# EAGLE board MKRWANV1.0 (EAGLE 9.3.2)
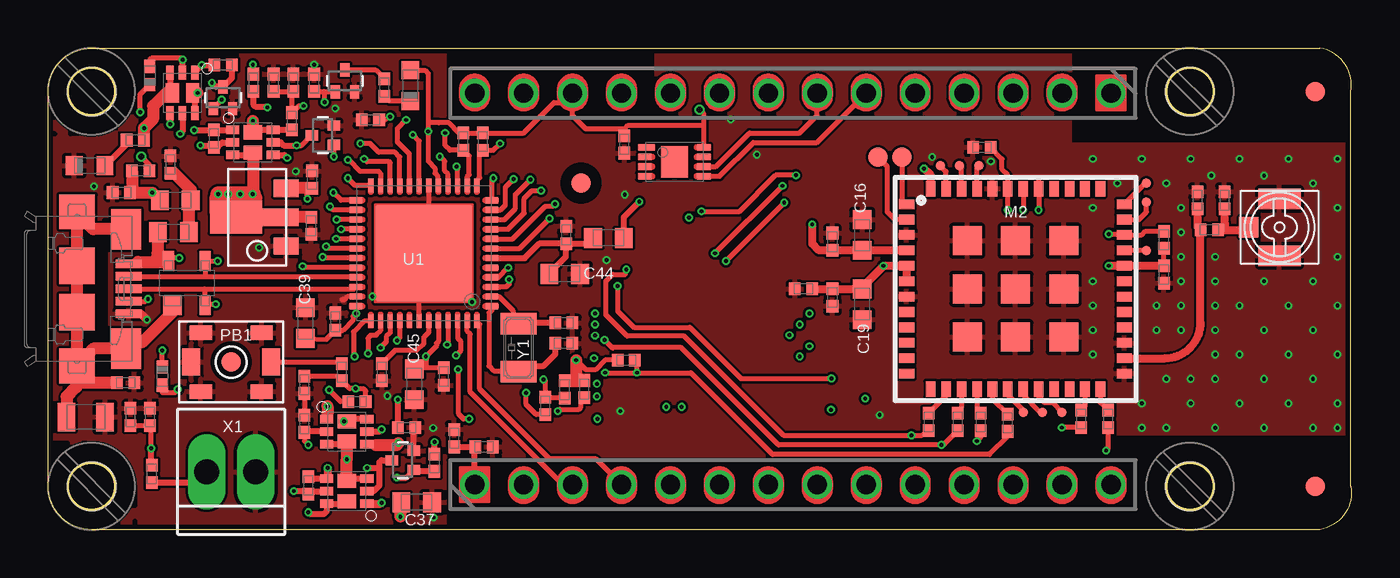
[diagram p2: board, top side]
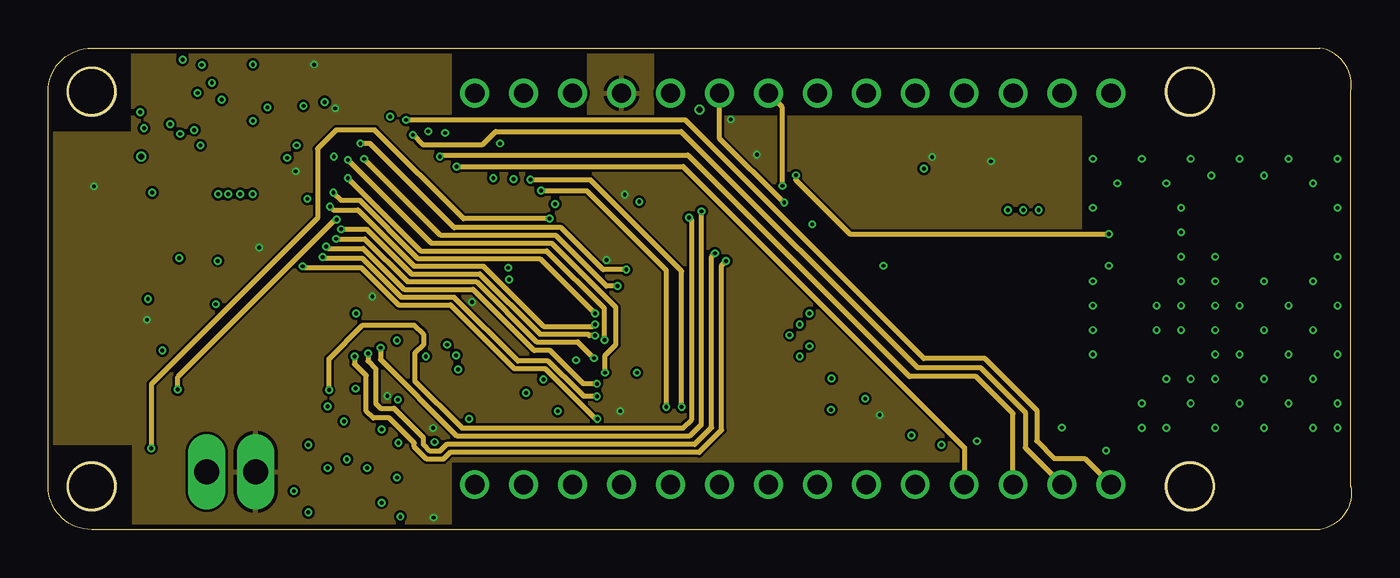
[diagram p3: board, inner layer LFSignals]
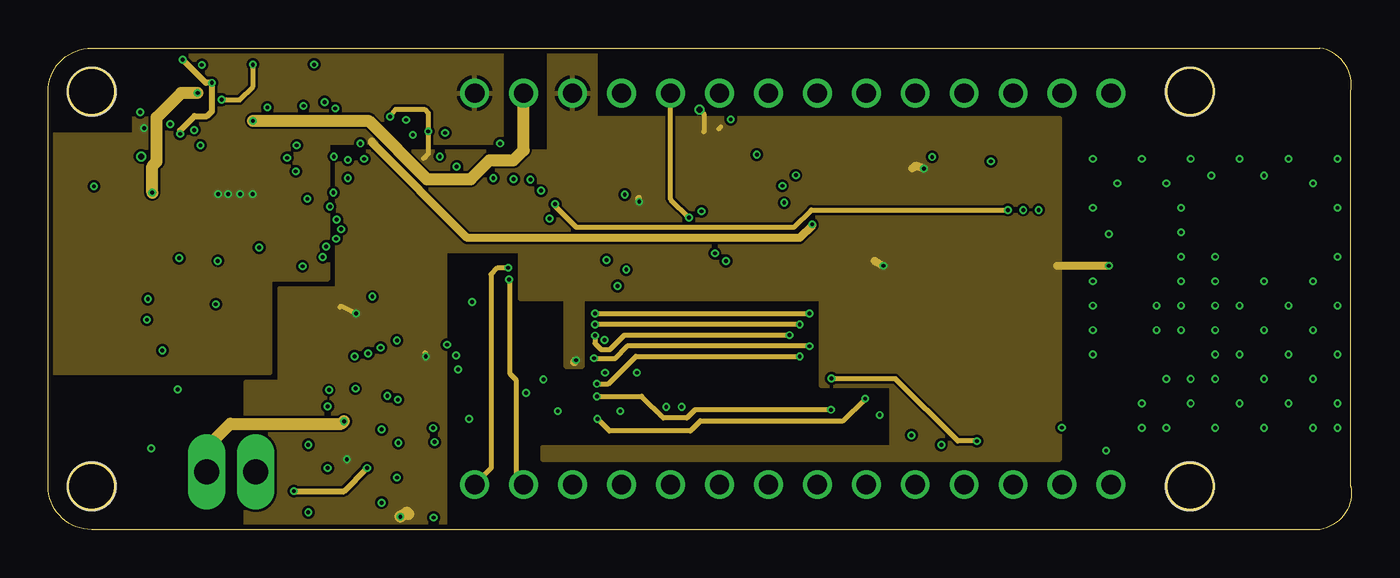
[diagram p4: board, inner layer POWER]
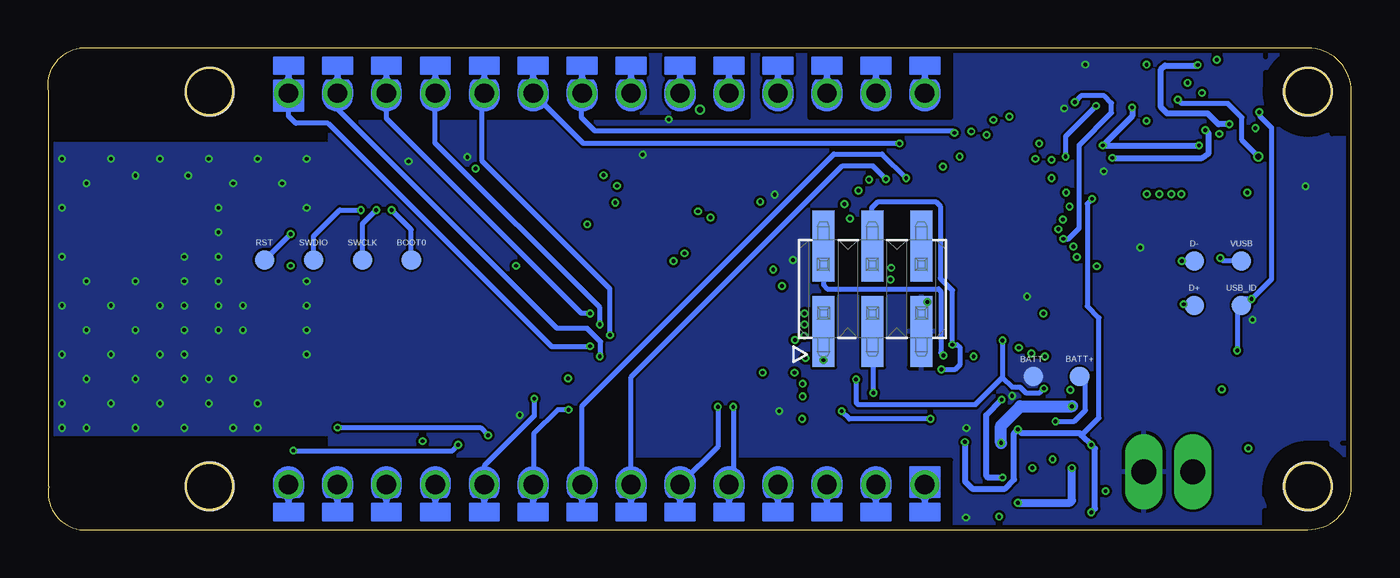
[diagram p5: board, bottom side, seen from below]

Size 67.63 x 25 mm. Coordinates in mm from the lower left corner, seen from the top.
Outline: 66,0 2.25,0 arc-90 0,2.25 0,22.75 arc-90 2.25,25 66,25 arc-90 67.6,22.75 67.6,2.25 arc-90 66,0
Copper layers (1*2*15*16): Top 0.035mm / dielectric 0.2mm / LFSignals 0.0175mm / dielectric 0.3mm / POWER 0.0175mm / dielectric 0.2mm / Bottom 0.035mm
Design rules "B&B_4layers *": minimum track width 8mil, minimum drill 0.195mm, track to track 5mil, track to pad 5mil, pad to pad 5mil, via to via 5mil, smd to smd 0mil, copper to edge 10mil, drill to drill 8mil, minimum pad ring 6mil, minimum via ring 4mil, stop-mask expansion 4mil, vias tented up to drill 25mil, thermal gap 7mil
Net classes: 0 default: width 0.25 mm, drill 0.195 mm
Holes 2.5 mm at 2.25,2.25 2.25,22.75 59.25,22.75 59.25,2.25
tRestrict: area 0,0 to 4.5,4.5; area 0,20.5 to 4.5,25; 18 lines
bRestrict: area 0,0 to 4.5,4.5; area 0,20.5 to 4.5,25; 18 lines

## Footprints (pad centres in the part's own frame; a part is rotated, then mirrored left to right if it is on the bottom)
TP-1.00MM = smd 1 x 1 bottom: X 0,0
0805-R2013X50N = smd 0.95 x 1.45: 1 -1,0; 2 1,0
0402-1005X55N = smd 0.62 x 0.62: 1 -0.45,0; 2 0.45,0
0603-1608X90N = smd 0.95 x 1: 1 -0.8,0; 2 0.8,0
SOT190P230X110-4N = smd 1 x 1: 1 -1.15,0.75 | smd 1 x 0.6: 2 -1.15,-0.95; 3 1.15,-0.95; 4 1.15,0.95
SODFL1008X40N-882D = smd 0.65 x 0.6: A 0.475,0; C -0.475,0
LEDC1608X80N-AK = smd 0.9 x 0.95: A 0.8,0; C -0.8,0
FD-1-1.5 = smd 1.016 x 1.016: P$1 0,0
ZX62-AB-5PA = smd 0.4 x 1.35: 1 -1.3,3.025; 2 -0.65,3.025; 3 0,3.025; 4 0.65,3.025; 5 1.3,3.025 | smd 2.1 x 1.6: 6 3.1,2.9; 11 -3.1,2.9 | smd 1.8 x 1.9: 7 4,0.35; 10 -4,0.35 | smd 1.9 x 1.9: 8 1.2,0.35; 9 -1.2,0.35
2X3_SMT = smd 1.143 x 3.683: 1 -2.54,-2.223; 2 -2.54,2.223; 3 0,-2.223; 4 0,2.223; 5 2.54,-2.223; 6 2.54,2.223
1X14_SMD_TH = drill 1: 1 0,0; 2 2.54,0; 3 5.08,0; 4 7.62,0; 5 10.16,0; 6 12.7,0; 7 15.24,0; 8 17.78,0; 9 20.32,0; 10 22.86,0; 11 25.4,0; 12 27.94,0; 13 30.48,0; 14 33.02,0
U.FL-R-SMT-1(60) = smd 1.05 x 2.2: GND1 -1.475,0; GND2 1.475,0 | smd 1.05 x 1: SIG 0,-1.6
0603-1608X90N@1 = smd 0.95 x 1: 1 -0.8,0; 2 0.8,0
CMWX1ZZABZ-078 = smd 0.8 x 0.5: 1 -5.65,4.4; 2 -5.65,3.6; 3 -5.65,2.8; 4 -5.65,2; 5 -5.65,1.2; 6 -5.65,0.4; 7 -5.65,-0.4; 8 -5.65,-1.2; 9 -5.65,-2; 10 -5.65,-2.8; 11 -5.65,-3.6; 12 -5.65,-4.4; 25 5.65,-4.4; 26 5.65,-3.6; 27 5.65,-2.8; 28 5.65,-2; 29 5.65,-1.2; 30 5.65,-0.4; 31 5.65,0.4; 32 5.65,1.2; 33 5.65,2; 34 5.65,2.8; 35 5.65,3.6; 36 5.65,4.4 | smd 0.5 x 0.8: 13 -4.4,-5.2; 14 -3.6,-5.2; 15 -2.8,-5.2; 16 -2,-5.2; 17 -1.2,-5.2; 18 -0.4,-5.2; 19 0.4,-5.2; 20 1.2,-5.2; 21 2,-5.2; 22 2.8,-5.2; 23 3.6,-5.2; 24 4.4,-5.2; 37 4.4,5.2; 38 3.6,5.2; 39 2.8,5.2; 40 2,5.2; 41 1.2,5.2; 42 0.4,5.2; 43 -0.4,5.2; 44 -1.2,5.2; 45 -2,5.2; 46 -2.8,5.2; 47 -3.6,5.2; 48 -4.4,5.2 | smd 1.5 x 1.5: 49 -2.5,2.5; 50 0,2.5; 51 2.5,2.5; 52 -2.5,0; 53 0,0; 54 2.5,0; 55 -2.5,-2.5; 56 0,-2.5; 57 2.5,-2.5
C&K_PTS820_NO_HOLES = smd 1.15 x 0.75: 1 -1.575,1.525; 2 -1.575,-1.525; 3 1.575,1.525; 4 1.575,-1.525 | smd 0.95 x 1.4: 5 -2.075,0; 6 2.075,0
PWR_SC70 = smd 0.69 x 0.4: D1 1.04,0.65; D2 -1.04,-0.65; G1 -1.04,0; G2 1.04,0; S1 -1.04,0.65; S2 1.04,-0.65 | smd 1 x 0.7: D1' 0,0.525; D2' 0,-0.525
SOTFL50P160X78-3 = smd 0.5 x 0.66: D 0,0.57; G -0.5,-0.57; S 0.5,-0.57
TP-0.50MM = smd 0.5 x 0.5 bottom: X 0,0
QFN50P700X700X90-49XN-EPSQ515 = smd 0.65 x 0.28: 1 -3.525,2.75; 2 -3.525,2.25; 3 -3.525,1.75; 4 -3.525,1.25; 5 -3.525,0.75; 6 -3.525,0.25; 7 -3.525,-0.25; 8 -3.525,-0.75; 9 -3.525,-1.25; 10 -3.525,-1.75; 11 -3.525,-2.25; 12 -3.525,-2.75; 25 3.525,-2.75; 26 3.525,-2.25; 27 3.525,-1.75; 28 3.525,-1.25; 29 3.525,-0.75; 30 3.525,-0.25; 31 3.525,0.25; 32 3.525,0.75; 33 3.525,1.25; 34 3.525,1.75; 35 3.525,2.25; 36 3.525,2.75 | smd 0.28 x 0.65: 13 -2.75,-3.525; 14 -2.25,-3.525; 15 -1.75,-3.525; 16 -1.25,-3.525; 17 -0.75,-3.525; 18 -0.25,-3.525; 19 0.25,-3.525; 20 0.75,-3.525; 21 1.25,-3.525; 22 1.75,-3.525; 23 2.25,-3.525; 24 2.75,-3.525; 37 2.75,3.525; 38 2.25,3.525; 39 1.75,3.525; 40 1.25,3.525; 41 0.75,3.525; 42 0.25,3.525; 43 -0.25,3.525; 44 -0.75,3.525; 45 -1.25,3.525; 46 -1.75,3.525; 47 -2.25,3.525; 48 -2.75,3.525 | smd 5 x 5: 49 0,0
SOT89-3L = smd 0.9 x 1.3: 1 -1.5,0; 3 1.5,0 | smd 0.9 x 1.9: 2 0,0.3 | smd 1.7 x 2.7: TH 0,2.6
SON50P300X200X60-9N-EP160X140 = smd 0.85 x 0.3: 1 -1.45,0.75 | smd 0.7 x 0.3: 2 -1.525,0.25; 3 -1.525,-0.25; 4 -1.525,-0.75; 5 1.525,-0.75; 6 1.525,-0.25; 7 1.525,0.25; 8 1.525,0.75 | smd 1.4 x 1.6: 9 0,0
SCREW2 = drill 1.3 long: GND 1.27,0; V+ -1.27,0
ABS07 = smd 1.1 x 1.9: 1 -1.25,0; 2 1.25,0

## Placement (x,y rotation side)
BATT+  DNP  [TP-1.00MM]  14.1,7.96 0 top
BATT-  DNP  [TP-1.00MM]  16.5,7.95 0 top
BOOT0  DNP  [TP-1.00MM]  48.78,14 0 top
C1  4n7  [0805-R2013X50N]  1.95,5.85 0 top
C2  10n  [0402-1005X55N]  6.35,18.95 90 top
C3  100n  [0402-1005X55N]  13.3,7.53 270 top
C4  20p  [0402-1005X55N]  26.76,9.67 180 top
C5  20p  [0402-1005X55N]  26.76,10.73 180 top
C6  100n  [0402-1005X55N]  3.8,17.5 180 top
C7  4u7  [0402-1005X55N]  21.07,4.75 90 top
C8  100n  [0402-1005X55N]  4.28,5.85 90 top
C9  100n  [0402-1005X55N]  22.62,4.3 0 top
C10  DNP  [0402-1005X55N]  59.64,17.1 90 top
C11  100n  [0402-1005X55N]  29.9,20 270 top
C12  DNP  [0402-1005X55N]  61.04,17.1 90 top
C14  100n  [0402-1005X55N]  11.7,23.2 90 top
C15  1u  [0402-1005X55N]  13.65,15.78 270 top
C16  10u  [0603-1608X90N]  42.25,15.3 90 top
C17  1u  [0402-1005X55N]  13.7,18.18 90 top
C18  100n  [0402-1005X55N]  40.7,14.95 90 top
C19  10u  [0603-1608X90N]  42.25,11.7 270 top
C20  1u  [0402-1005X55N]  40.7,12.05 270 top
C21  100n  [0402-1005X55N]  39.2,12.5 180 top
C22  100n  [0402-1005X55N]  57.9,13.25 270 top
C37  10u  [0603-1608X90N]  19.12,1.43 0 top
C38  100n  [0402-1005X55N]  16.73,21.27 180 top
C39  10u  [0603-1608X90N]  13.35,10.72 90 top
C40  100n  [0402-1005X55N]  14.9,10.8 90 top
C42  100n  [0402-1005X55N]  20.52,7.95 270 top
C43  100n  [0402-1005X55N]  26.88,15.3 90 top
C44  10u  [0603-1608X90N]  26.81,13.28 0 top
C45  10u  [0603-1608X90N]  19,7.55 270 top
C47  1u  [0402-1005X55N]  17.32,8.18 270 top
D1  PRTR5V0U2X,215  [SOT190P230X110-4N]  7.2,12.8 90 top
D1+  DNP  [TP-1.00MM]  44.3,19.35 0 bottom
D1-  DNP  [TP-1.00MM]  43.05,19.35 0 bottom
D2  PMEG2005EL  [SODFL1008X40N-882D]  5.92,7.97 270 top
D3  PMEG2005EL  [SODFL1008X40N-882D]  5.28,23.57 90 top
D+  DNP  [TP-1.00MM]  8.15,11.65 0 top
D-  DNP  [TP-1.00MM]  8.15,13.95 0 top
DL1  YELLOW  [LEDC1608X80N-AK]  18.8,23.05 90 top
DL2  GREEN  [LEDC1608X80N-AK]  2.15,18.9 0 top
F1  PTC  [0603-1608X90N]  6.5,15.45 180 top
FD1  DNP  [FD-1-1.5]  27.65,18 90 top
FD2  DNP  [FD-1-1.5]  65.75,22.75 180 top
FD3  DNP  [FD-1-1.5]  65.75,2.25 90 top
FD4  DNP  [FD-1-1.5]  9.5,8.7 0 top
FRAME1  DNP  [FRAME]  0,0 0 top
FRAME2  DNP  [FRAME]  0,0 0 top
J1  USB-MICRO  [ZX62-AB-5PA]  1.15,12.5 270 top
J2  DNP  [2X3_SMT]  24.85,12.5 0 bottom
J3  DNP  [1X14_SMD_TH]  22.13,2.34 0 top
J5  DNP  [1X14_SMD_TH]  55.15,22.66 180 top
J7  UFL  [U.FL-R-SMT-1(60)]  63.9,15.7 270 top
L1  FERRITE-470R  [0603-1608X90N@1]  6.6,17.1 180 top
L5  FERRITE-470R  [0603-1608X90N@1]  29.07,15.14 180 top
M2  CMWX1ZZABZ-078  [CMWX1ZZABZ-078]  50.2,12.5 0 top
PB1  RESET  [C&K_PTS820_NO_HOLES]  9.5,8.7 0 top
Q1  DMP2160UFDB  [PWR_SC70]  6.97,22.68 270 top
Q2  DMP2160UFDB  [PWR_SC70]  10.62,20.1 0 top
Q3  2N7002T  [SOTFL50P160X78-3]  14.25,20.48 90 top
Q4  2N7002T  [SOTFL50P160X78-3]  9.07,22.43 0 top
Q5  DMP2160UFDB  [PWR_SC70]  15.5,2 180 top
Q6  DMP2160UFDB  [PWR_SC70]  15.5,5.1 0 top
Q7  2N7002T  [SOTFL50P160X78-3]  18.4,3.6 90 top
Q8  2N7002T  [SOTFL50P160X78-3]  15.4,23.3 0 top
R1  1M  [0402-1005X55N]  4.03,7.62 180 top
R2  330R  [0402-1005X55N]  25.8,6.42 90 top
R3  330R  [0402-1005X55N]  15.25,8.18 270 top
R4  10k  [0402-1005X55N]  27.82,7.3 90 top
R5  10k  [0402-1005X55N]  26.8,7.28 90 top
R6  330R  [0402-1005X55N]  16.02,6.65 180 top
R7  330R  [0402-1005X55N]  17.45,22.95 270 top
R8  330k  [0402-1005X55N]  5.28,5.85 270 top
R9  680k  [0402-1005X55N]  5.38,2.9 270 top
R10  10k  [0402-1005X55N]  13.3,5.5 270 top
R11  10k  [0402-1005X55N]  13.5,2.3 90 top
R12  100k  [0402-1005X55N]  18.6,5.3 180 top
R13  47k  [0402-1005X55N]  20.05,3.48 90 top
R14  10k  [0402-1005X55N]  30,8.8 180 top
R16  10k  [0402-1005X55N]  57.9,15.05 270 top
R17  10k  [0402-1005X55N]  48.45,19.85 0 top
R18  DNP  [0402-1005X55N]  45.7,5.6 270 top
R19  DNP  [0402-1005X55N]  47.2,5.6 270 top
R20  0R  [0402-1005X55N]  48.4,5.6 270 top
R21  4k7  [0402-1005X55N]  21.55,20.15 90 top
R22  4k7  [0402-1005X55N]  22.55,20.15 90 top
R23  100k  [0402-1005X55N]  12.65,21.2 270 top
R24  100k  [0402-1005X55N]  12.72,23.2 270 top
R25  100k  [0402-1005X55N]  4.8,18.62 180 top
R26  330R  [0402-1005X55N]  10.65,23.2 90 top
R27  10k  [0402-1005X55N]  9.07,24.12 180 top
R28  10k  [0402-1005X55N]  8.6,20.3 90 top
R29  330R  [0402-1005X55N]  4.53,20.23 0 top
R30  0R  [0402-1005X55N]  60.26,15.56 0 top
R31  0R  [0402-1005X55N]  49.8,5.55 270 top
R32  0R  [0402-1005X55N]  53.6,5.75 270 top
R33  100k  [0402-1005X55N]  13.8,23.2 270 top
R34  0R  [0402-1005X55N]  55,5.75 270 top
RST  DNP  [TP-1.00MM]  56.4,14 0 top
SWCLK  DNP  [TP-1.00MM]  51.32,14 0 top
SWDIO  DNP  [TP-1.00MM]  53.86,14 0 top
TP1  DNP  [TP-0.50MM]  51.6,6.1 0 bottom
TP2  DNP  [TP-0.50MM]  50.6,6.1 0 bottom
TP3  DNP  [TP-0.50MM]  57,18 0 bottom
TP4  DNP  [TP-0.50MM]  57,17 0 bottom
TP5  DNP  [TP-0.50MM]  46.3,18.9 0 bottom
TP6  DNP  [TP-0.50MM]  47.3,18.9 0 bottom
TP7  DNP  [TP-0.50MM]  48.3,18.9 0 bottom
TP15  DNP  [TP-0.50MM]  57,14.5 0 bottom
TP18  DNP  [TP-0.50MM]  52.6,6.1 0 bottom
U1  D21G18  [QFN50P700X700X90-49XN-EPSQ515]  19.5,14.35 180 top
U2  LDO2SOT89-3L  [SOT89-3L]  12.35,16.23 90 top
U3  ECC508  [SON50P300X200X60-9N-EP160X140]  32.5,19.1 0 top
U$5  [MH_RND_F_2.2MM_NM]  2.25,2.25 90 top
U$6  [MH_RND_F_2.2MM_NM]  2.25,22.75 90 top
U$7  [MH_RND_F_2.2MM_NM]  59.25,22.75 90 top
U$8  [MH_RND_F_2.2MM_NM]  59.25,2.25 90 top
USB_ID  DNP  [TP-1.00MM]  5.7,11.65 0 top
VUSB  DNP  [TP-1.00MM]  5.7,13.95 0 top
X1  SCREW2X2.54  [SCREW2]  9.5,3 0 top
Y1  32.768KHz  [ABS07]  24.42,9.44 270 top

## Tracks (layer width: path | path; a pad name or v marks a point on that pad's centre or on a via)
+3V3  (via drill 0.2, 0.3)
  Top 0.25: 15.35,3.8 v15.5,3.65 | 20.8,21.12 20.27,21.12
  Top 0.254: 20.25,10.45 U1.44 20.25,9.78 20.15,9.68 20.15,9.55 v19.6,9 19.6,8.4 | 20.25,18.1 U1.17 20.23,18.32 20.07,18.5 20.07,18.75 19.73,19.12 v19.73,20.68 19.73,21.2 | U1.36 v15.97,11.22 15.82,11.07 15.82,10.88 15.3,10.35 C40.1 14.43,9.88 C39.1 | C42.1 19.6,8.4 | 19.6,8.4 C45.1 | DL1.A 19.55,23.85 19.73,23.68 19.73,21.2 | C38.1 17.48,21.27 v17.75,21.45 | 20.8,21.12 21.32,20.6 R21.2 R22.2 24.68,20.6 26.25,22.18 26.73,22.18 J5.12 27.2,22.64 27.2,21.5 27.9,20.8 29.9,20.8 | R14.2 28.9,8.8 28.4,8.3 27.9,8.3 v27.4,8.8 | C22.1 R16.2 | U3.8 34.02,21 | 34.02,21 34.02,21.57 v33.8,21.8 | C11.1 29.9,20.8 | 29.9,20.8 30.1,21 34.02,21 | 20.27,21.12 19.8,21.12 19.73,21.2
  Top 0.305: Q5.D2 15.62,2.65 Q5.D2' | Q6.D2 15.38,4.45 Q6.D2' | L5.1 29.87,16.22 v30.68,17.02
  Top 0.406: M2.6 M2.5 v43.35,13.7 42.3,12.65 C19.1 C20.1 C21.1 | M2.48 45.8,18.4 v45.45,18.75 | v55.05,13.7 M2.32 C22.1
  Top 0.61: v27.4,8.8 27.4,7.75 27.35,7.72 | Q5.D2' v15.5,3.65 Q6.D2' | R5.2 27.35,7.72 | 27.35,7.72 27.8,7.72 R4.2 | C37.1 v18.27,0.68
  POWER 0.254: 19.48,19.27 19.73,19.52 v19.73,20.68 19.73,21.62 19.52,21.82 18.02,21.82 v17.75,21.45 | v15.97,11.22 15.2,11.6 15.15,11.55 | v19.6,9 19.6,9.12 19.55,9.18 | 34.8,20.8 34.9,20.9 | v33.8,21.8 34.02,21.57 34.02,20.65
  POWER 0.305: v30.68,17.02 30.62,17.2 30.65,17.23
  POWER 0.406: 27.3,8.7 v27.4,8.8 | v43.35,13.7 42.95,13.9 42.9,13.95 | v45.45,18.75 45,18.9 44.85,18.75 | v55.05,13.7 52.35,13.7
  POWER 0.61: v18.27,0.68 18.62,0.88 18.7,0.8
  Bottom 0.254: v27.4,8.8 27.4,10.27 J2.1
  pour POWER: 52.5,21.35 28.4,21.35 28.4,24.9 26,24.9 26,19.6 15,19.6 15,12.5 12,12.5 12,7.65 10.25,7.65 10.25,0.05 20.6,0.05 20.6,14.5 24.5,14.5 24.5,12 26.85,12 26.85,8.47 27.72,8.47 27.72,12 40.1,12 40.1,7.5 43.75,7.5 43.75,4.25 25.65,4.25 25.65,3.65 52.5,3.65
+5V  (via drill 0.2)
  Top 0.25: 8.7,17.55 v8.82,17.43
  Top 0.254: U2.TH U2.2
  Top 0.305: Q2.D2 10.5,19.45 Q2.D2' | Q1.D2 6.33,22.8 Q1.D2'
  Top 0.406: M2.4 C16.1 C18.1 40,14.5 39.65,14.85 v39.65,15.85
  Top 0.61: R29.2 v4.97,20.85 5.45,21.32 5.45,22 6.12,22.68 Q1.D2' | U2.TH 10.51,16.23 10.79,16.51 10.79,17.23 v10.61,17.43 10.62,17.45 Q2.D2' | 10.62,17.43 10.62,17.4 | 8.75,16.4 8.7,16.4 8.7,17.3 v8.82,17.43 | C15.1 U2.2
  Top 0.813: v8.82,17.43 v10.61,17.43 10.62,17.43
  POWER 0.406: 16.8,20.15 16.8,20.1 21.75,15.15 39,15.15 39.65,15.8 v39.65,15.85
  other vias: 9.34,17.43 9.97,17.43
  pour POWER: 23.5,25 23.5,20.1 14.5,20.1 14.5,13 11.5,13 11.5,8.15 0,8.15 0,20.5 4.5,20.5 4.5,25
GND  (via drill 0.2)
  Top 0.254: U1.18 19.75,14.6 U1.49 19.25,14.1 U1.42 | U1.35 15.53,12.1 15.38,11.95 15.28,11.95 15.25,11.93 | C3.2 R10.1
  Top 0.305: Q7.S 18.97,5.22 R12.1
  Top 0.406: J1.5 4.83,11.2 v5.12,10.9
  other vias: 43.15,5.95 56.75,6.55 58.02,7.82 66.91,9.09 60.56,5.28 58.02,5.28 63.1,5.28 65.64,5.28 66.91,5.28 28.98,14 29.93,17.4 16.82,12.1 22,11.82 10.95,14.65 19.98,5.28 20,0.62 12.85,18.6 14.9,21.88 13.8,24.15 2.38,17.82 36.77,19.48 17.6,6.94 45.88,19.35 48.92,19.12 60.56,10.36 65.64,10.36 54.21,11.63 54.21,16.71 54.21,19.25 55.48,17.98 56.75,19.25 58.02,17.98 60.36,18.38 63.1,18.38 65.64,17.98 59.29,19.25 61.83,19.25 64.37,19.25 66.91,19.25 66.91,16.71 66.91,14.17 60.56,12.9 60.56,14.17 63.1,12.9 65.64,12.9 61.83,11.63 64.37,11.63 66.91,11.63 63.1,10.36 61.83,9.09 64.37,9.09 65.64,7.82 63.1,7.82 60.56,7.82 59.29,6.55 61.83,6.55 64.37,6.55 66.91,6.55 29.69,6.15 58.79,12.9 58.79,14.17 58.79,10.36 58.79,11.63 59.29,7.82 57.52,10.36 57.52,11.63 60.56,11.63 58.79,15.44 58.79,16.71 54.21,10.36 54.21,9.09 54.21,12.9 60.56,9.09 56.75,5.28 35.42,21.3
  pour Bottom: 52.85,20 67.6,20 67.6,5 52.85,5
  pour Top: -1,25 53,25 53,0 -1,0
  pour Bottom: -1,25 53,25 53,0 -1,0
  pour Top (isolate 0.1): 52.88,20 67.6,20 67.6,5 52.88,5
  pour LFSignals: 0,4.5 0,20.55 4.45,20.55 4.45,25 20.8,25 20.8,21 28.1,21 28.1,25 31.3,25 31.3,21.4 53.52,21.4 53.52,5 53.52,3.6 20.8,3.6 20.8,0 4.5,0 4.5,4.5
N1  (via drill 0.2)
  Top 0.305: Q5.S2 13.6,2.65 R11.2
  Top 0.406: Q5.S1 17.25,1.35 v17.3,1.4 | v14.5,3.2 14.5,2.69 Q5.S2
  Bottom 0.406: v17.3,1.4 14.6,1.4 14.5,1.5 v14.5,3.2
N2  (via drill 0.2)
  Top 0.305: 13.65,2 R11.1 | Q5.G1 16.9,2 17.2,2.3 17.2,3.2 | 17.2,3.2 17.2,3.5 17.3,3.6 Q7.D | 13.65,2 v12.75,2 | v16.55,3.2 17.2,3.2 | 13.65,2 Q5.G2
  POWER 0.305: v12.75,2 15.35,2 v16.55,3.2
N3  (via drill 0.2)
  Top 0.305: v18.1,2.7 18.57,2.7 Q7.G 19.05,3.02 R13.1 | R12.2 v18.15,6.75
  Bottom 0.305: v18.1,2.7 18.85,2.7 18.95,2.8 18.95,5.95 v18.15,6.75
N17650912  (via drill 0.2)
  Top 0.25: v6.8,14.1 6.4,14.1 D1.4
  Top 0.254: J1.1 4.55,13.8 4.65,13.9
  Top 0.61: 6,13.95 D1.4 6.2,13.9 5.75,13.9 | 4.65,13.9 5.45,13.9 | 5.45,13.9 5.75,13.9 | VUSB.X 5.75,13.9 | F1.2 5.65,14.1 5.45,13.9
  Bottom 0.25: VUSB.X 6.65,13.95 v6.8,14.1
N17658775
  Top 0.254: PB1.6 15.18,8.7 R3.1
N17690335  (via drill 0.2)
  Top 0.305: Q1.S2 v6.33,21.05 | R27.2 v7.97,24.12 7.62,23.77 Q1.S1
  Bottom 0.305: v6.33,21.05 6.9,21.05 7.45,21.6 9.55,21.6 9.88,21.93 9.88,23.9 9.68,24.1 8,24.1 v7.97,24.12
N17690346  (via drill 0.2)
  Top 0.254: D3.A 5.28,24.4 5.38,24.5 6.88,24.5 v6.97,24.4
  Top 0.305: R27.1 9.53,23.45 Q4.D 8.71,23 v8.5,23.2 | 7,21.61 Q1.G2 6.97,20.68 v6.85,20.55 | Q1.G1 v6.97,24.4
  POWER 0.305: v6.97,24.4 8.18,23.2 v8.5,23.2 8.5,21.73 8.25,21.48 7.6,21.48 6.85,20.73 v6.85,20.55
N17690381  (via drill 0.2, 0.3)
  Top 0.254: R25.1 5.28,18.62 5.28,18.93 v4.83,19.38 | v10.62,24.15 10.62,23.68 R26.2 | Q4.G 8.57,21.9 v9,22.32
  POWER 0.254: v9,22.32 9.95,22.32 10.62,23 v10.62,24.15
  Bottom 0.254: v4.83,19.38 5.67,20.23 5.67,21.4 6.4,22.12 8.8,22.12 v9,22.32
N17690821  (via drill 0.2)
  Top 0.305: Q2.S1 R28.2 v7.58,20.75 | Q2.S2 12.25,19.45 v12.4,19.3
  Bottom 0.305: v12.4,19.3 7.75,19.3 7.4,19.55 7.4,20.57 v7.58,20.75
N17690840  (via drill 0.2)
  Top 0.254: v12.9,19.95 13.15,19.95 Q3.D
  Top 0.305: Q2.G1 9.05,20.1 8.8,19.85 R28.1 8.5,19.95 v7.9,19.95 | Q2.G2 12.07,20.1 12.22,19.95 v12.9,19.95 | R26.1 10.65,22.07 10.75,21.98 11.32,21.98 v11.38,21.93
  Bottom 0.305: v7.9,19.95 v12.9,19.95 11.38,21.48 v11.38,21.93
N17690878  (via drill 0.2)
  Top 0.254: C14.1 R24.2 12.65,22.68 R23.1 13,22 v13.25,22 | Q3.G v14.82,19.38
  Bottom 0.254: v14.82,19.38 14.82,20.43 v13.25,22
N17834267
  Top 0.305: 2.95,19.15 DL2.A 4.08,20.02 R29.1
N17852357
  Top 0.305: C43.1 27.98,14.85 L5.2 | U1.6 24.73,14.1 25.48,14.85 C43.1 | C44.1 25.98,13.28 26.88,14.18 C43.1
N$1
  Top 0.61: 6.5,11.6 D1.1 6.45,11.3 4.88,9.72 4.33,9.72 J1.6 2.35,9.4 J1.7 | J1.7 J1.8 J1.9 J1.10 2.35,15.6 J1.11 | J1.7 1.46,7.53 | 1.46,7.53 1.46,7.4 0.95,6.89 C1.1 | R1.2 1.56,7.62 1.46,7.53
N$2
  Top 0.61: F1.1 7.35,17.05 L1.1 7.4,17.65 6.55,18.5 C2.1
N$3
  Top 0.254: DL1.C 17.7,22.25 R7.2
N$4  (via drill 0.2)
  Top 0.254: v24.8,7.1 24.8,6.5 25.32,5.97 R2.1
  Bottom 0.254: v24.8,7.1 24.8,10.23 J2.3
N$5
  Top 0.254: M2.24 54.6,6.6 R34.1
N$6
  Top 0.254: Q8.D 16.98,23.87 R7.1
N$7
  Top 0.254: M2.23 53.8,6.4 R32.1
N$8  (via drill 0.2)
  Top 0.254: v13.45,17.18 13.45,17.48 C17.1 | R10.2 13.3,4.6 v13.5,4.4
  Top 0.305: Q6.G1 13.55,5.1 R10.2 | v13.5,0.9 13.6,0.8 14.3,0.8 14.46,0.96 Q5.D1 15.38,1.35 Q5.D1' 15.3,1.27 | Q6.G2 17.2,5.1 v17.3,5.2 | R13.2 v20.05,4.55
  Top 0.61: C17.1 U2.3
  Bottom 0.254: v13.45,17.18 13.7,16.93 13.7,11.6 13.1,11 13.1,5.8 14,4.9
  Bottom 0.305: v17.3,5.2 17.1,5 14.1,5 14,4.9 v13.5,4.4 13.3,4.2 13.3,1.1 v13.5,0.9 | v20.05,4.55 20.05,2.5 19.68,2.12 17.98,2.12 17.5,2.6 17.5,5 v17.3,5.2 | 17.27,5.17 v17.3,5.2
N$9
  Top 0.254: TP1.X 51.5,6.1 50.6,7 M2.19
N$10
  Top 0.254: M2.14 46.6,6.95 R18.1
N$11
  Top 0.254: M2.15 47.4,6.35 R19.1
N$12  (via drill 0.2)
  Top 0.254: Q6.S1 14.46,5.86 14.5,5.9 v14.5,6.4
  Top 0.305: Q6.S2 16.95,4.45 17,4.4
  Top 0.61: 17,4.4 18.1,4.4 v18.18,4.5 | v14.5,6.4 14.5,6
  Bottom 0.61: v18.18,4.5 18.18,5.4 17.18,6.4 v14.5,6.4
N$13
  Top 0.254: M2.16 48.2,6.35 R20.1
N$14
  Top 0.254: M2.17 49,6.8 R31.1
N$15  (via drill 0.2)
  Top 0.254: v51.4,16.6 M2.41 51.4,18.15
  Bottom 0.254: SWDIO.X 53.86,15.24 52.5,16.6 v51.4,16.6
N$16  (via drill 0.2)
  Top 0.254: M2.42 v50.6,16.6
  Bottom 0.254: SWCLK.X 51.32,15.88 v50.6,16.6
N$17
  Top 0.406: R30.2 61.2,15.56 | 61.2,15.56 62.3,15.56 J7.SIG | C12.1 61.04,15.96 61.05,15.95 61.05,15.71 61.2,15.56
N$18
  Top 0.254: D1+.X 44.3,17.15 M2.1
N$19
  Top 0.254: M2.2 43.95,16.1 43.55,16.5 43.55,18.85 D1-.X
N$20
  Top 0.254: M2.18 49.8,7 50.6,6.2 TP2.X
N$21
  Top 0.254: TP3.X 56.95,18 M2.36
N$22
  Top 0.254: M2.35 56.6,16.1 57,16.5 TP4.X
N$23
  Top 0.254: M2.47 46.6,18.6 TP5.X
N$24
  Top 0.254: M2.46 47.4,18.8 TP6.X
N$25
  Top 0.254: M2.45 48.2,18.8 TP7.X
N$33
  Top 0.254: TP15.X M2.33
N$36
  Top 0.254: M2.20 51.4,6.9 51.7,6.6 52.1,6.6 TP18.X
N$38
  Top 0.406: 59.81,15.6 R30.1 | C10.1 59.64,15.73 R30.1 | M2.26 57.95,8.9 arc90 59.8,10.75 R30.1 arc-90 R30.1
N$46
  Top 0.254: U1.43 19.75,10.25 19.5,10 19.5,9.65 19.15,9.35 19.12,9.32 18.02,9.32 C47.1
PA00_XIN32
  Top 0.254: U1.1 23.02,11.4 22.88,11.25 22.88,8.5 23.12,8.25 24.16,8.25 Y1.2 24.54,8.51
  Top 0.305: 24.54,8.51 25.71,8.51 26.31,9.11 C4.2
PA01_XOUT32
  Top 0.254: U1.2 23.4,12.1 24.12,11.38 24.12,10.79 Y1.1
  Top 0.305: C5.2 24.26,10.73 Y1.1
PA02_AIN0  (via drill 0.2)
  Top 0.254: 23.48,12.6 U1.3 23.77,12.6 23.93,12.75 v23.93,12.99
  POWER 0.254: J3.2 24.27,2.74 24.27,7.78 23.98,8.07 23.98,12.93 v23.93,12.99
PA03_VREFA  (via drill 0.2)
  Top 0.254: U1.4 23.38,13.1 v23.88,13.6
  Top 0.305: C7.1 C9.1 22.14,4.26 J3.1
  POWER 0.254: v23.88,13.6 23.32,13.6 22.98,13.25 22.98,3.18 J3.1
PA04_AIN4  (via drill 0.2)
  Top 0.254: U1.9 23.88,15.6 24.7,16.43 24.7,17.2 25.1,17.6 v25.57,17.6
  LFSignals 0.254: v25.57,17.6 27.95,17.6 32.08,13.47 v32.08,6.38
  Bottom 0.254: v32.08,6.38 32.08,2.56 J3.5
PA05_AIN5  (via drill 0.2)
  Top 0.254: U1.10 23.68,16.1 24.25,16.68 24.25,17.4 v25.02,18.18
  LFSignals 0.254: v25.02,18.18 28.12,18.18 32.88,13.43 v32.88,6.38
  Bottom 0.254: 34.88,2.38 J3.6 32.88,4.3 v32.88,6.38
PA06_AIN6  (via drill 0.2)
  Top 0.254: 23.95,18 v24.15,18.2 23.73,17.77 23.73,16.85 23.48,16.6 U1.11 23.38,16.6
  Bottom 0.254: v24.15,18.2 24.85,18.9 26.4,18.9 37.38,7.92 J3.7
PA07_AIN7  (via drill 0.2)
  Top 0.254: U1.12 23.02,18.12 v23.1,18.25
  Bottom 0.254: 39.95,2.38 J3.8 39.91,6.43 26.85,19.5 24.35,19.5 v23.1,18.25
PA08_S0_I2C_SDA  (via drill 0.2)
  Top 0.254: v23.45,20.05 23.1,19.7 R22.1 22.4,19.55 22.4,18.27 22.25,18.12 U1.13 | J5.6 39.9,20.1 36.6,20.1 34.85,18.35 U3.5
  Bottom 0.254: J5.6 39.84,20.05 v23.45,20.05
PA09_S0_I2C_SCL  (via drill 0.2)
  Top 0.254: 21.75,19.5 R21.1 | R21.1 20.85,19.7 20.6,19.95 v20.6,20.6 | 21.82,19.43 R21.1 | 21.75,18.15 21.75,18.32 21.85,18.43 21.85,19.4 R21.1 | J5.7 39.9,22.64 39.9,21.5 39,20.6 36.4,20.6 34.65,18.85 U3.6
  Top 0.305: 21.75,18.15 U1.14
  Bottom 0.254: J5.7 39.95,22.62 39.95,21.4 39.25,20.7 20.7,20.7 v20.6,20.6
PA10_TCC0-W2  (via drill 0.2)
  Top 0.254: U1.15 21.25,18.75 v21.2,18.85
  LFSignals 0.254: v21.2,18.85 32.95,18.85 47.55,4.25 47.55,2.35 J3.11
PA11_TCC0-W3  (via drill 0.2)
  Top 0.254: U1.16 20.75,18.45 20.57,18.62 20.57,19.12 v20.32,19.38 20.5,19.2
  LFSignals 0.254: 20.3,19.4 v20.32,19.38 20.35,19.4 20.35,19.45 33.2,19.45 44.7,7.95 48.15,7.95 50.08,6.03 J3.12
PA12_MOSI_TX  (via drill 0.2)
  Top 0.254: v30,13.5 29.95,13.25 29.3,13.25 28.95,12.9 28.95,11.15 30.05,10.05 33,10.05 38.15,4.9 v44.8,4.9 45.35,4.9 R18.2 | U1.21 18.25,19.35 18,19.6 17.15,19.6 16.7,20.05 v16.2,20.05 | R32.2 v52.6,5.3
  LFSignals 0.254: v16.2,20.05 16.7,20.05 21.07,15.68 26.62,15.68 28.8,13.5 v30,13.5
  Bottom 0.254: v52.6,5.3 45.2,5.3 v44.8,4.9
PA13_SCK  (via drill 0.2)
  Top 0.254: U1.22 17.75,19.05 17.7,19.1 16.55,19.1 v16.4,19.25 | v40.65,7.85 35.95,7.85 33.3,10.5 30.4,10.5 29.55,11.35 v29.55,12.65 | R20.2 48.4,4.8 v48.2,4.6
  LFSignals 0.254: v29.55,12.65 28.98,12.65 26.35,15.28 20.38,15.28 v16.4,19.25
  POWER 0.254: v48.2,4.6 47.2,4.6 43.95,7.85 v40.65,7.85
PA14_RF_SSN  (via drill 0.2)
  Top 0.254: v15.55,19.2 15.6,19.2 16.2,18.6 17.15,18.6 17.25,18.5 U1.23 | v28.9,8.15 v30.55,8.15 | v30.55,8.15 33.35,8.15 37.6,3.9 48.85,3.9 49.8,4.85 R31.2 | v30.55,8.15 30.55,8.7 R14.1
  LFSignals 0.254: v28.9,8.15 28.9,9.05 29.45,9.6 29.45,11.55 26.12,14.88 19.88,14.88 v15.55,19.2 15.6,19.2
  Bottom 0.254: 30.6,8.1 v30.55,8.15
PA15_MISO_RX  (via drill 0.2)
  Top 0.254: U1.24 15.93,17.88 v15.55,18.25 | v28.88,9.85 29.3,9.43 29.32,9.45 32.85,9.45 37.9,4.4 v46.35,4.4 46.45,4.4 R19.2 | R34.2 55,4.2 v54.9,4.1
  LFSignals 0.254: v15.55,18.25 19.32,14.47 25.88,14.47 28.85,11.5 28.85,9.88 v28.88,9.85
  Bottom 0.254: v54.9,4.1 46.65,4.1 v46.35,4.4
PA16_S1_MOSI  (via drill 0.2)
  Top 0.254: U1.25 15.2,17.1 v14.8,17.5
  LFSignals 0.254: v14.8,17.5 15.2,17.1 16.15,17.1 19.18,14.07 25.52,14.07 v28.38,11.22
  POWER 0.254: v28.38,11.22 v39.5,11.22
  Bottom 0.254: 50.17,22.12 50.17,22.56 J5.3 | v39.5,11.22 39.95,11.22 50.08,21.35 J5.3 | J5.3
PA17_S1_SCK  (via drill 0.2)
  Top 0.254: U1.26 14.8,16.6 v14.62,16.77
  LFSignals 0.254: v14.62,16.77 14.8,16.6 16.07,16.6 19,13.68 22.57,13.68 25.7,10.55 28.27,10.55 v28.38,10.65
  POWER 0.254: v39,10.65 v28.38,10.65
  Bottom 0.254: J5.4 47.55,22.64 47.55,20.07 39,11.53 v39,10.65
PA18_USB_ID  (via drill 0.2)
  Top 0.254: U1.27 v14.97,16.1 | 5.92,7.12 6,7.12 | 6,7.12 6.58,7.12 v6.72,7.28 | D2.A 5.92,7.2 6,7.12
  LFSignals 0.254: v14.97,16.1 14.9,16.1 6.72,7.92 v6.72,7.28
PA19_S1_MISO  (via drill 0.2)
  Top 0.254: U1.28 v15.2,15.6
  LFSignals 0.254: v15.2,15.6 16.52,15.6 18.82,13.3 18.82,13.28 22.4,13.28 25.52,10.15 28,10.15 28.07,10.07 v28.38,10.07
  POWER 0.254: v28.38,10.07 28.38,9.68 28.7,9.35 29.15,9.35 29.9,10.1 v38.48,10.1
  Bottom 0.254: v38.48,10.1 38.48,12.5 45.1,19.12 45.1,22.55 J5.5
PA20_TCC0-W6  (via drill 0.2)
  Top 0.254: R33.2 14.3,22.75 | 14.3,22.75 14.88,22.75 Q8.G | v14.35,22.2 14.35,22.7 14.3,22.75 | U1.29 v14.95,15.1
  LFSignals 0.254: v14.95,15.1 16.43,15.1 18.65,12.88 22.23,12.88 25.35,9.75 27.48,9.75 v28.32,8.9
  POWER 0.254: v39.5,9.53 30.05,9.53 29.4,8.88 28.35,8.88 v28.32,8.9
  Bottom 0.254: v14.95,15.1 14.68,15.1 14.12,15.65 14.12,19.98 12.45,21.65 12.45,22.15 12.82,22.52 14.03,22.52 v14.35,22.2 | J5.1 55.15,21.48 54.77,21.1 53.1,21.1 41.5,9.5 39.52,9.5 v39.5,9.53
PA21_TCC0-W7  (via drill 0.2)
  Top 0.254: U1.30 14.53,14.6 v14.43,14.7
  LFSignals 0.254: v14.43,14.7 14.53,14.6 16.35,14.6 18.48,12.47 22.05,12.47 25.23,9.3 26.05,9.3 27.77,7.58 v28.48,7.58
  POWER 0.254: v39,9 30.5,9 29.07,7.58 v28.48,7.58
  Bottom 0.254: v39,9 39.05,9 38.95,9.1 38.95,9.75 39.65,10.45 41.23,10.45 52.7,21.93 52.7,22.57 J5.2
PA22_TC4-W0  (via drill 0.2)
  Top 0.254: U1.31 14.3,14.1 v14.25,14.15
  LFSignals 0.254: v14.25,14.15 14.28,14.15 14.32,14.1 16.3,14.1 18.32,12.07 21.05,12.07 24.38,8.75 25.95,8.75 27.55,7.17 27.8,6.92 v28.48,6.92
  POWER 0.254: v40.62,6.22 33.58,6.22 33.15,5.8 31.93,5.8 30.8,6.92 v28.48,6.92
  Bottom 0.254: v40.62,6.22 41.17,6.22 42.42,4.97 42.42,2.37 J3.9
PA23_TC4-W1  (via drill 0.2)
  Top 0.254: U1.32 13.28,13.6 v13.2,13.68
  LFSignals 0.254: v13.2,13.68 13.28,13.6 16.25,13.6 18.18,11.68 20.88,11.68 24.2,8.35 25.8,8.35 28.4,5.75 v28.5,5.75
  POWER 0.254: v42.4,6.8 41.25,5.65 33.85,5.65 33.33,5.12 29.12,5.12 v28.5,5.75
  Bottom 0.254: 45.02,2.37 J3.10 45,3.3 42.4,5.9 v42.4,6.8
PA27_RF_NRES  (via drill 0.2)
  Top 0.254: U1.39 17.75,10.22 17.55,10.03 17.55,9.75 v17.25,9.45 | v55.05,15.35 55.8,15.35 M2.34 56.75,15.3 56.95,15.5 R16.1 | v33.9,16.52 35.88,16.52 37.75,18.4 v38.8,18.4
  LFSignals 0.254: v17.25,9.45 17.25,8.82 21.23,4.85 33.27,4.85 33.9,5.47 v33.9,16.52 | v55.05,15.35 41.6,15.35 38.8,18.15 v38.8,18.4
  Bottom 0.254: RST.X v55.05,15.35
PA30_SWCLK  (via drill 0.2)
  Top 0.254: U1.45 20.75,9.65 v20.7,9.6 | v21.85,5.75 21.55,5.75 21.3,6 21.3,8.3 v21.27,8.32 | 27.85,6.83 R4.1 27.65,6.67 27.65,6.35 27.55,6.25 26.55,6.25 v26.45,6.15
  Bottom 0.254: J2.4 24.9,14.77 24.9,16.7 24.6,17 21.52,17 21.32,16.8 21.32,13.05 20.7,12.43 v20.7,9.6 20.45,9.6 20.32,9.47 20.32,8.55 20.57,8.3 21.25,8.3 v21.27,8.32 | v21.85,5.75 26.05,5.75 v26.45,6.15
PA31_SWDIO  (via drill 0.2)
  Top 0.254: U1.46 21.25,9.95 21.4,9.8 21.4,9.28 v21.18,9.05
  Bottom 0.254: J2.2 27.39,12.69 27.2,12.5 21.43,12.5 21.3,12.38 21.3,9.18 v21.18,9.05
PB02_AIN10
  Top 0.254: J3.3 27.16,2.4 26.6,2.4 26.6,2.45 21.9,7.15 21.9,10.15 21.75,10.3 U1.47
PB03_AIN11
  Top 0.25: J3.4 29.41,2.34
  Top 0.254: U1.48 22.4,10.68 22.4,7.3 26,3.7 28.39,3.7 J3.4
PB08_AIN3  (via drill 0.2)
  Top 0.254: U1.7 24.48,14.6 v26.02,16.15 | v5.35,4.22 5.35,5.33 R8.2 C8.1
  Top 0.305: R9.1 5.35,3.35 v5.35,4.22
  LFSignals 0.254: v26.02,16.15 21.55,16.15 16.95,20.75 14.95,20.75 13.97,19.77 13.97,16.18 5.35,7.55 v5.35,4.22
PB09_BOOT0  (via drill 0.2)
  Top 0.254: v49.8,16.6 M2.43 49.8,18.4 49.5,18.7 49.5,19.25 R17.2 | U1.8 24.1,15.1 25.8,16.8 26.2,16.8 v26.3,16.9
  POWER 0.254: v26.3,16.9 26.3,16.8 27.4,15.7 38.7,15.7 39.6,16.6 v49.8,16.6
  Bottom 0.254: BOOT0.X 48.78,15.58 v49.8,16.6
PB10_TCC0-W4  (via drill 0.2)
  Top 0.254: U1.19 19.25,20.18 v18.93,20.5
  LFSignals 0.254: v18.93,20.5 19.43,20 22.55,20 23.23,20.68 32.85,20.68 45.12,8.4 48.4,8.4 50.7,6.1 50.7,4.25 J3.13
PB11_TCC0-W5  (via drill 0.2)
  Top 0.254: U1.20 18.75,19.5 18.12,20.12 18.12,20.82 v18.57,21.27
  LFSignals 0.254: v18.57,21.27 33.05,21.27 45.44,8.89 45.45,8.9 48.6,8.9 51.3,6.2 51.3,4.6 52.2,3.7 53.8,3.7 J3.14
PB22_S5_TX  (via drill 0.2)
  Top 0.254: U1.37 16.4,10.82 15.85,10.28 15.85,9.05 v15.9,9 | v35.17,13.95 v38.2,16.98
  LFSignals 0.254: 35,13.78 v35.17,13.95 34.95,13.72 34.95,5.17 33.77,4 20.85,4 20.5,3.65 19.65,3.65 19,4.3 19,4.5 17.7,5.8 16.88,5.8 16.5,6.15 16.5,8 15.9,8.6 v15.9,9 | v38.2,16.98 38.17,16.98 34.85,20.3 34.85,22.64 J5.9
PB23_S5_RX  (via drill 0.2)
  Top 0.254: 17.25,10.47 U1.38 17.25,10.32 17.02,10.1 16.75,10.1 16.6,9.95 v16.6,9.15 | v34.6,14.35 v38.1,17.85
  LFSignals 0.254: v16.6,9.15 16.6,8.75 17,8.35 17,6.55 17.25,6.3 17.95,6.3 19.48,4.78 19.48,4.42 19.82,4.08 20.32,4.08 20.68,4.42 33.55,4.42 34.42,5.3 34.42,14.18 v34.6,14.35 | v38.1,17.85 38.1,21.93 J5.8
RESET#  (via drill 0.2)
  Top 0.254: J5.10 | R6.2 15.18,6.65 v14.57,7.25
  LFSignals 0.254: v33.25,16.2 33.4,16.05 33.4,5.72 32.95,5.28 21.48,5.28 19.02,7.72 19.02,9.15 19.48,9.6 19.48,10.15 19,10.62 16.32,10.62 14.57,8.88 v14.57,7.25
  POWER 0.254: v33.25,16.2 32.3,17.15 J5.10
RESETN  (via drill 0.2)
  Top 0.254: v25.7,7.8 25.8,7.7 R2.2 26.7,6.88 R5.1 | U1.40 18.25,9.97 v18.1,9.82 | 15.28,7.7 R3.2 | R6.1 16.48,7.2 16.35,7.33 v15.95,7.33 15.65,7.33 R3.2 | C3.1 15,7.97 R3.2
  Bottom 0.254: v25.7,7.8 25.7,6.6 25.6,6.5 19.5,6.5 18.1,7.9 | v18.1,9.82 18.1,7.9 | 18.1,7.9 17.6,7.4 17.2,7.4 16.9,7.1 16.18,7.1 v15.95,7.33
USB_ID  (via drill 0.2)
  Top 0.254: J1.4 5.05,11.85 v5.17,11.97 | D2.C v5.92,9.3 | v4.78,21.68 4.78,22.6 D3.C
  Bottom 0.254: v5.92,9.3 5.92,11.7 5.65,11.97 v5.17,11.97 4.15,13 4.15,20.88 4.78,21.5 v4.78,21.68
  Bottom 0.305: USB_ID.X 5.5,11.65 v5.17,11.97
USB_N  (via drill 0.2)
  Top 0.25: J1.2 8.1,13.15 | 8.1,13.15 8.15,13.2 D-.X v8.8,13.95 | 8.1,13.15 16,13.15 15.97,13.12 U1.33
  Bottom 0.25: v8.8,13.95 8.2,13.9 D-.X
USB_P  (via drill 0.2)
  Top 0.25: J1.3 8.1,12.5 | 8.1,12.5 8.15,12.45 D+.X 8.2,11.7 v8.7,11.7 | 8.1,12.5 15.9,12.5 15.97,12.57 U1.34
  Bottom 0.25: D+.X 8.65,11.65 v8.7,11.7
VBATT  (via drill 0.2)
  Top 0.305: Q6.D1 15.62,5.75 Q6.D1' | R9.2 7.68,2.45 X1.V+
  Top 0.61: Q6.D1' v15.35,5.62
  POWER 0.61: v15.35,5.62 15.22,5.5 9.45,5.5 8.53,4.58 8.53,3.25 8.48,3.25 X1.V+
  Bottom 0.254: v15.35,5.62 14.38,5.62 13.8,6.2 13.8,7.66 BATT+.X
VIN  (via drill 0.2)
  Top 0.305: R23.2 Q2.D1 10.75,20.75 Q2.D1'
  Top 0.61: Q2.D1' v10.62,21.23
  POWER 0.61: v10.62,21.23 16.62,21.23 19.65,18.2 21.93,18.2 22.9,19.18 24.15,19.18 24.68,19.7 J5.13 | J5.13
VUSB  (via drill 0.2)
  Top 0.305: 4.25,18.52 R25.2 | Q1.D1 7.62,22.55 Q1.D1'
  Top 0.61: L1.2 v5.4,17.5 C6.1 4.35,17.6 R25.2 | Q1.D1' v7.75,22.68
  POWER 0.406: 5.45,17.45 v5.4,17.5
  POWER 0.61: v7.75,22.68 6.9,22.68 5.62,21.4 5.62,19.1 5.4,18.88 v5.4,17.5

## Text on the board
tPlace: PB1
tNames: X1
